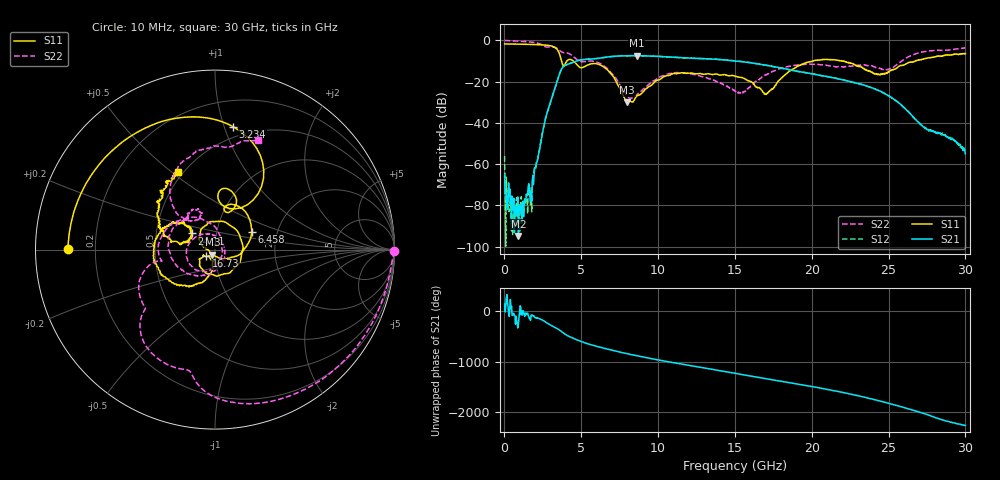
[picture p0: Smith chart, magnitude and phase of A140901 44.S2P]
!  2-Port S-parameters saved by WinCal
! VAR MeasName=S-Parameters (CALIBRATED_DATA) read from VNA (N5244A)
! VAR MeasDate=11/3/2014 9:34:03 AM
! VAR NAME=A140901 44
! VAR FILENAME=A140901 44.S2P
! VAR DATE=11/3/2014 9:34:03 AM
! VAR PHYS_PORTS=1,2
# Hz S RI R 50
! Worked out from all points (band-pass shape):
!   801 points, 10 MHz to 30 GHz, reference 50 ohm
!   highest |S21| = -7.40 dB at 8.595 GHz (marker M1); lowest = -94.9 dB at 909.7 MHz (marker M2)
!   |S21| within 3 dB of the highest: 4.541 GHz to 15.58 GHz (11.04 GHz wide, 110 % of centre)
!   lowest |S11| = -30.0 dB at 7.995 GHz (marker M3), VSWR 1.07, Z = 48.5 - j2.75 ohm
!   |S11| at or under -10 dB: 3.715 GHz to 4.065 GHz (350.6 MHz wide, 9.01 % of centre); 4.481 GHz to 20.11 GHz (15.63 GHz wide, 127 % of centre); 22 GHz to 26.73 GHz (4.73 GHz wide, 19.4 % of centre)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
!   |S22| runs from -28.3 to 0.0 dB; largest |S21 - S12| = 0.0031
!   S11 on the Smith chart (normalised r, x): 10 MHz: 0.10, +0.00; 3.234 GHz: 0.41, +1.07; 6.458 GHz: 1.47, +0.31; 16.73 GHz: 0.90, -0.07; 24.11 GHz: 0.76, +0.14; 30 GHz: 0.47, +0.52
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1e7  -0.8189 0.00206  -0.000461 0.000283  0.00152 -0.000359  0.9964 -0.00986
1.974375e8  -0.8153 0.0652  -7.81e-05 1.69e-05  -7.31e-05 -2.08e-05  0.9748 -0.1313
9.097e8  -0.7566 0.2902  -9.3e-06 1.54e-05  -6.28e-05 3.23e-05  0.7992 -0.5279
1.621962e9  -0.6271 0.4961  -0.000203 -0.000158  -0.000202 -0.000135  0.4545 -0.7998
2.634125e9  -0.2782 0.7189  -0.0101 0.00421  -0.0101 0.0043  -0.1292 -0.6956
3.233925e9  0.1 0.6851  0.0358 0.0466  0.0356 0.0465  -0.3376 -0.5908
4.021162e9  0.0158 0.2997  -0.0732 -0.2447  -0.0728 -0.2447  -0.4083 -0.2878
5.033325e9  0.0612 0.2084  -0.1544 0.3021  -0.1548 0.3016  -0.2964 -0.065
6.45785e9  0.2037 0.1004  0.3777 -0.0655  0.3778 -0.0641  -0.171 0.1712
7.994838e9  -0.0144 -0.0283  -0.2148 -0.3657  -0.2139 -0.366  0.0377 0.0235
8.594638e9  -0.0448 0.0011  -0.3989 -0.1517  -0.3986 -0.1522  0.0389 -0.025
1.001916e10  -0.0899 0.0641  -0.1791 0.3692  -0.1783 0.368  -0.0375 -0.1189
1.219344e10  0.1289 0.096  0.3698 -0.00428  0.3693 -0.0032  -0.1517 0.0208
1.365545e10  0.0922 -0.1186  0.0763 -0.3419  0.078 -0.343  -0.0646 0.0843
1.5005e10  -0.0593 -0.1216  -0.272 -0.1647  -0.2731 -0.1646  0.0371 0.0458
1.672942e10  -0.0501 -0.0374  -0.1283 0.2282  -0.1278 0.2272  -0.0121 -0.1277
1.837888e10  -0.0406 -0.1515  0.1676 0.1098  0.1676 0.1113  -0.2087 -0.0965
2.002832e10  -0.2671 -0.162  0.0936 -0.1223  0.0947 -0.1228  -0.2451 0.0915
2.411446e10  -0.1277 0.0902  0.0456 0.0478  0.0457 0.0484  -0.0839 0.2101
2.501416e10  -0.1635 0.0412  0.0409 -0.0188  0.0409 -0.0186  -0.1145 0.1641
2.662612e10  -0.285 0.0985  -0.013 -0.00402  -0.013 -0.00385  -0.2405 0.386
3e10  -0.2084 0.4299  -0.000351 -0.00173  -0.000701 -0.00203  0.2415 0.6126
